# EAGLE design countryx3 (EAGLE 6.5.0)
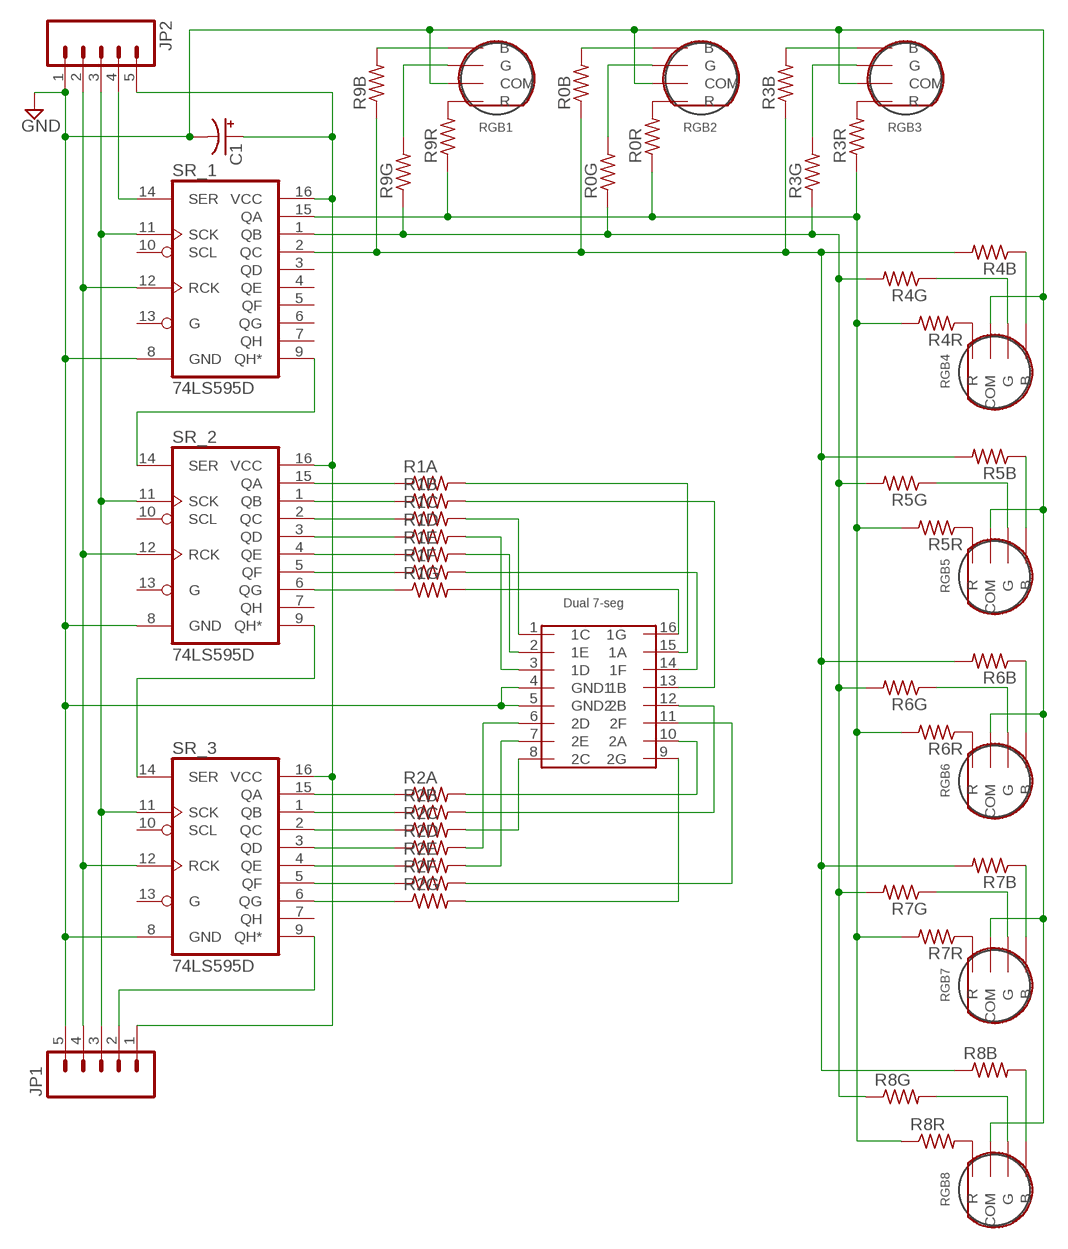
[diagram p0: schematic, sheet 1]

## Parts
C1  CPOL-USE2,5-6E  [E2,5-6E]
JP1  M05LOCK  [1X05_LOCK]
JP2  M05LOCK  [1X05_LOCK]
R0B  R-US_M0805  [M0805]
R0G  R-US_M0805  [M0805]
R0R  R-US_M0805  [M0805]
R1A  R-US_M0805  [M0805]
R1B  R-US_M0805  [M0805]
R1C  R-US_M0805  [M0805]
R1D  R-US_M0805  [M0805]
R1E  R-US_M0805  [M0805]
R1F  R-US_M0805  [M0805]
R1G  R-US_M0805  [M0805]
R2A  R-US_M0805  [M0805]
R2B  R-US_M0805  [M0805]
R2C  R-US_M0805  [M0805]
R2D  R-US_M0805  [M0805]
R2E  R-US_M0805  [M0805]
R2F  R-US_M0805  [M0805]
R2G  R-US_M0805  [M0805]
R3B  R-US_M0805  [M0805]
R3G  R-US_M0805  [M0805]
R3R  R-US_M0805  [M0805]
R4B  R-US_M0805  [M0805]
R4G  R-US_M0805  [M0805]
R4R  R-US_M0805  [M0805]
R5B  R-US_M0805  [M0805]
R5G  R-US_M0805  [M0805]
R5R  R-US_M0805  [M0805]
R6B  R-US_M0805  [M0805]
R6G  R-US_M0805  [M0805]
R6R  R-US_M0805  [M0805]
R7B  R-US_M0805  [M0805]
R7G  R-US_M0805  [M0805]
R7R  R-US_M0805  [M0805]
R8B  R-US_M0805  [M0805]
R8G  R-US_M0805  [M0805]
R8R  R-US_M0805  [M0805]
R9B  R-US_M0805  [M0805]
R9G  R-US_M0805  [M0805]
R9R  R-US_M0805  [M0805]
RGB1  RGBLED  [3LED]
RGB2  RGBLED  [3LED]
RGB3  RGBLED  [3LED]
RGB4  RGBLED  [3LED]
RGB5  RGBLED  [3LED]
RGB6  RGBLED  [3LED]
RGB7  RGBLED  [3LED]
RGB8  RGBLED  [3LED]
SR_1  74LS595D  [SO16]
SR_2  74LS595D  [SO16]
SR_3  74LS595D  [SO16]
U$1  HDSP-G03E  [HDSP-G]

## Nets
GND: C1.- JP1.5 JP2.1 RGB1.COM RGB2.COM RGB3.COM RGB4.COM RGB5.COM RGB6.COM RGB7.COM RGB8.COM SR_1.8(GND) SR_2.8(GND) SR_3.8(GND) U$1.4(GND1) U$1.5(GND2)
N$1: R0R.1 R3R.1 R4R.2 R5R.2 R6R.2 R7R.2 R8R.1 R9R.1 SR_1.15(QA)
N$2: R0B.1 R3B.1 R4B.2 R5B.2 R6B.2 R7B.2 R8B.1 R9B.1 SR_1.2(QC)
N$3: R8R.2 RGB8.R
N$4: R1G.2 U$1.16(1G)
N$5: R1F.2 U$1.14(1F)
N$6: R1C.2 U$1.1(1C)
N$7: R1G.1 SR_2.6(QG)
N$8: R9R.2 RGB1.R
N$9: R1A.2 U$1.15(1A)
N$10: R1B.2 U$1.13(1B)
N$11: R2B.2 U$1.12(2B)
N$12: R2F.2 U$1.11(2F)
N$13: R2B.1 SR_3.1(QB)
N$14: R2D.2 U$1.6(2D)
N$15: R2A.1 SR_3.15(QA)
N$16: R1D.1 SR_2.3(QD)
N$17: R2E.2 U$1.7(2E)
N$18: R0R.2 RGB2.R
N$19: R2C.1 SR_3.2(QC)
N$20: R3R.2 RGB3.R
N$21: R2A.2 U$1.10(2A)
N$22: R2D.1 SR_3.3(QD)
N$23: R2E.1 SR_3.4(QE)
N$24: R2F.1 SR_3.5(QF)
N$25: R9G.2 RGB1.G
N$26: R0G.2 RGB2.G
N$27: R3G.2 RGB3.G
N$28: R9B.2 RGB1.B
N$29: R0B.2 RGB2.B
N$30: R3B.2 RGB3.B
N$31: R2G.1 SR_3.6(QG)
N$32: R0G.1 R3G.1 R4G.2 R5G.2 R6G.2 R7G.2 R8G.1 R9G.1 SR_1.1(QB)
N$33: R1E.1 SR_2.4(QE)
N$34: R4G.1 RGB4.G
N$35: R4B.1 RGB4.B
N$36: R4R.1 RGB4.R
N$37: R2G.2 U$1.9(2G)
N$38: R1E.2 U$1.2(1E)
N$39: R5G.1 RGB5.G
N$40: R5B.1 RGB5.B
N$41: R5R.1 RGB5.R
N$42: R1F.1 SR_2.5(QF)
N$43: R6G.1 RGB6.G
N$44: R6B.1 RGB6.B
N$45: R6R.1 RGB6.R
N$46: R8G.2 RGB8.G
N$47: R8B.2 RGB8.B
N$48: R1D.2 U$1.3(1D)
N$49: R7G.1 RGB7.G
N$50: R7B.1 RGB7.B
N$51: R7R.1 RGB7.R
N$52: R2C.2 U$1.8(2C)
N$53: R1C.1 SR_2.2(QC)
N$54: R1B.1 SR_2.1(QB)
N$55: R1A.1 SR_2.15(QA)
RCLK: JP1.4 JP2.2 SR_1.12(RCK) SR_2.12(RCK) SR_3.12(RCK)
SCLK: JP1.3 JP2.3 SR_1.11(SCK) SR_2.11(SCK) SR_3.11(SCK)
SER_12: SR_1.9(QH*) SR_2.14(SER)
SER_23: SR_2.9(QH*) SR_3.14(SER)
SER_IN: JP2.4 SR_1.14(SER)
SER_OUT: JP1.2 SR_3.9(QH*)
VCC: C1.+ JP1.1 JP2.5 SR_1.16(VCC) SR_2.16(VCC) SR_3.16(VCC)
Unconnected: SR_1.3(QD) SR_1.4(QE) SR_1.5(QF) SR_1.6(QG) SR_1.7(QH) SR_1.10(SCL) SR_1.13(G) SR_2.7(QH) SR_2.10(SCL) SR_2.13(G) SR_3.7(QH) SR_3.10(SCL) SR_3.13(G)

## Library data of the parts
C1 = Power Supply:CPOL-US: POLARIZED CAPACITOR, American symbol
JP1 JP2 = SparkFun-Connectors:M05: Header 5 Standard 5-pin 0.1" header. Use with straight break away headers (SKU : PRT-00116), right angle break away headers (PRT-00553), swiss pins (PRT-00743), machine pins (PRT-00117), and female headers (PRT-00115). Molex polarized connector foot print use with SKU : PRT-08230 with associated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
R0B R0G R0R R1A R1B R1C R1D R1E R1F R1G R2A R2B R2C R2D R2E R2F R2G R3B R3G R3R R4B R4G R4R R5B R5G R5R R6B R6G R6R R7B R7G R7R R8B R8G R8R R9B R9G R9R = resistor:R-US_: RESISTOR, American symbol
RGB1-RGB8 = RISK:RGBLED
SR_1-SR_3 = SparkFun-DigitalIC:74*595: 8-bit SHIFT REGISTER, output latch; PROD_ID: IC-07875
U$1 = RISK:HDSP-G03E

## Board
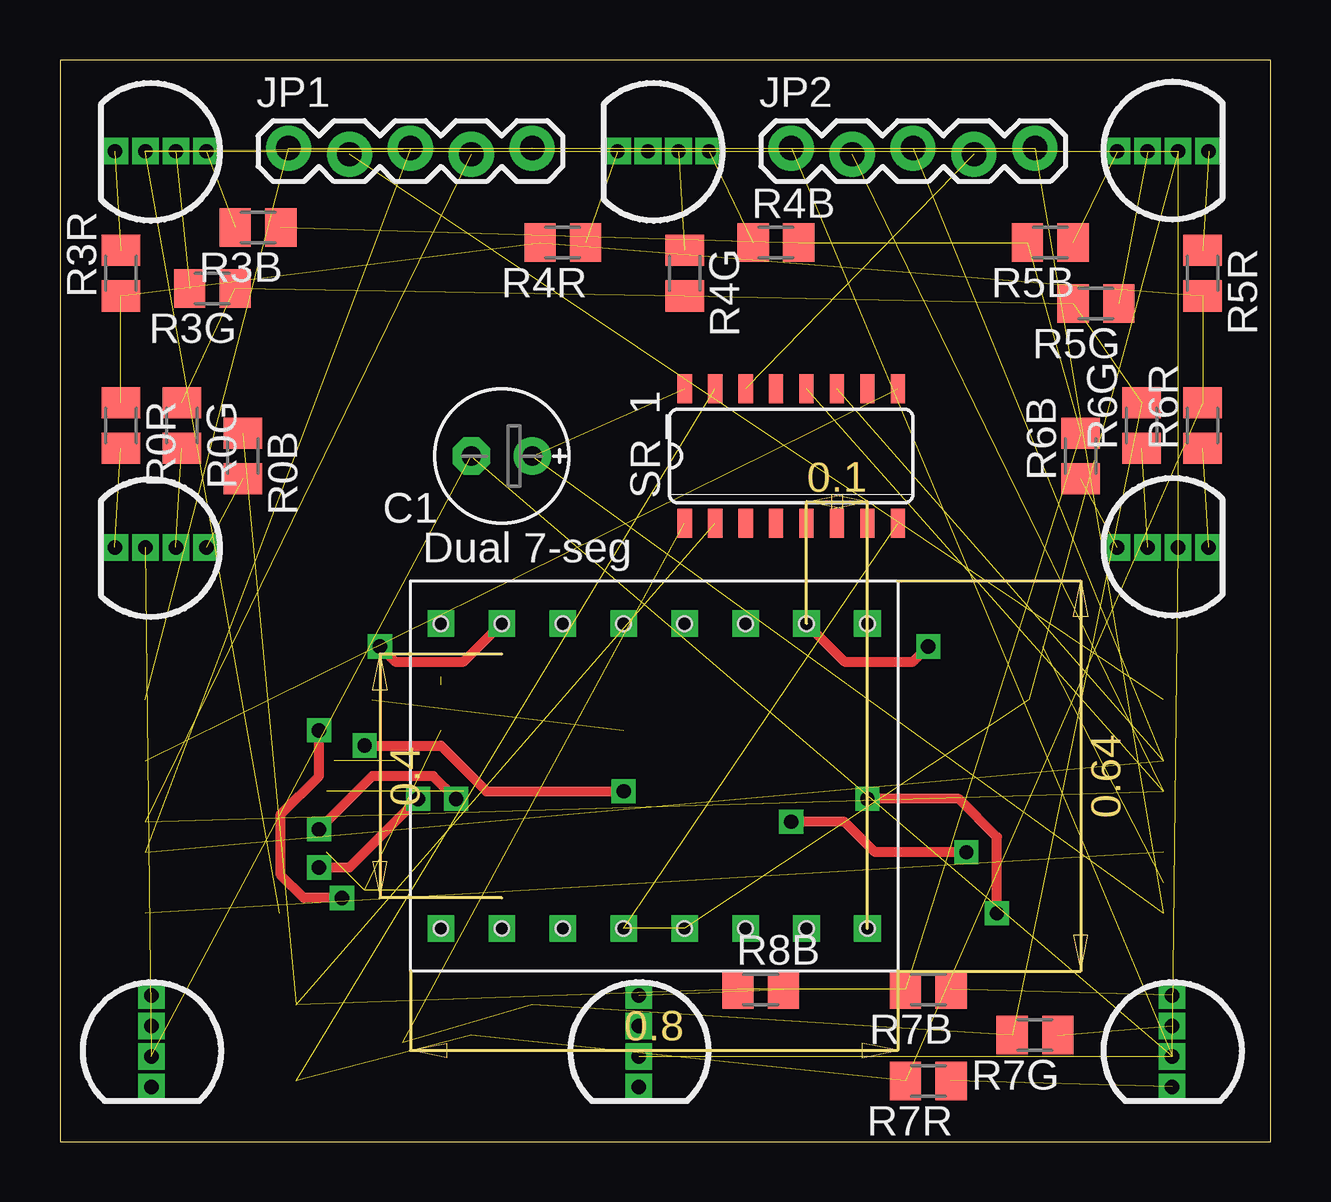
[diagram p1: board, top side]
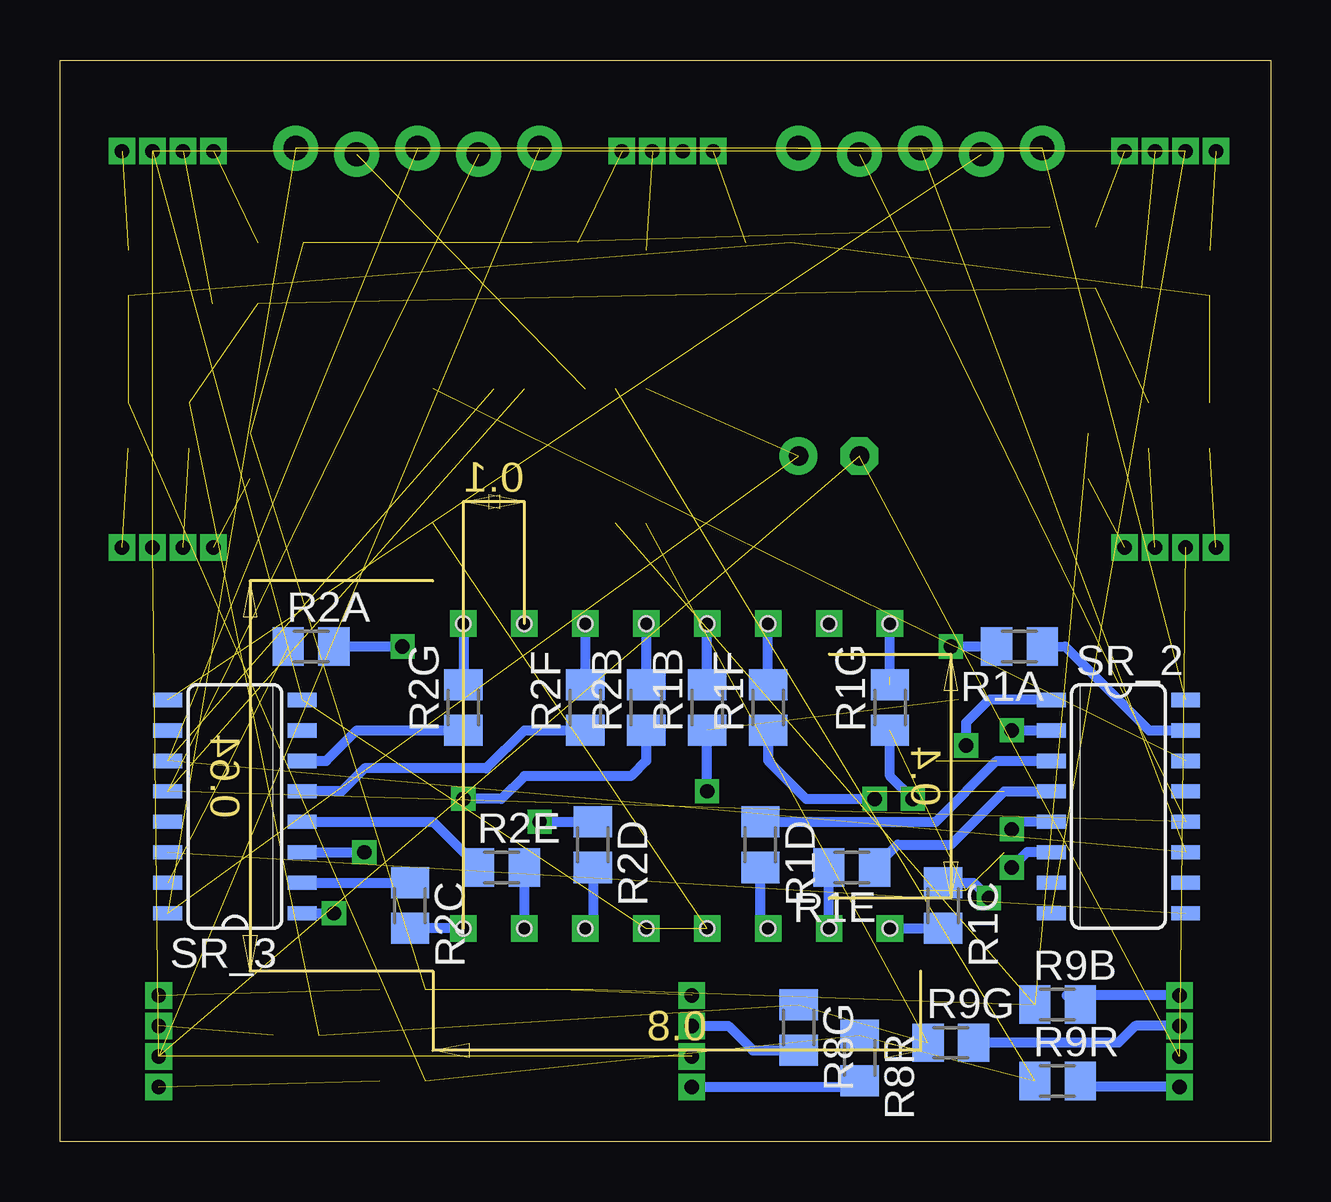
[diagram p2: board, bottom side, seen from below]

Size 50.47 x 45.08 mm. Coordinates in mm from the lower left corner, seen from the top.
Outline: 0,0 50.47,0 50.47,45.08 0,45.08 0,0
Copper layers (1*16): Top 0.035mm / dielectric 1.5mm / Bottom 0.035mm
Design rules "default": minimum track width 10mil, minimum drill 24mil, track to track 8mil, track to pad 8mil, pad to pad 8mil, via to via 8mil, smd to smd 8mil, copper to edge 40mil, drill to drill 8mil, minimum pad ring 10mil, minimum via ring 8mil, stop-mask expansion 4mil, vias tented up to drill 0mil, thermal gap 10mil

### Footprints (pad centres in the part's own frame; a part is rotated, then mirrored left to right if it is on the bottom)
E2,5-6E = drill 0.813 pad 1.575: + -1.27,0 | drill 0.813 pad 1.575 octagon: - 1.27,0
1X05_LOCK = drill 1.016 pad 1.88: 1 0,0.127; 2 2.54,-0.127; 3 5.08,0.127; 4 7.62,-0.127; 5 10.16,0.127
M0805 = smd 1.3 x 1.6: 1 -0.95,0; 2 0.95,0
3LED = drill 0.6 pad 0.61 square: B 0,2.286; COM 0,-0.254; G 0,1.016; R 0,-1.524
SO16 = smd 0.6 x 1.2: 1 -4.445,-2.8; 2 -3.175,-2.8; 3 -1.905,-2.8; 4 -0.635,-2.8; 5 0.635,-2.8; 6 1.905,-2.8; 7 3.175,-2.8; 8 4.445,-2.8; 9 4.445,2.8; 10 3.175,2.8; 11 1.905,2.8; 12 0.635,2.8; 13 -0.635,2.8; 14 -1.905,2.8; 15 -3.175,2.8; 16 -4.445,2.8
HDSP-G = drill 0.6 square: 1 -8.89,-6.35; 2 -6.35,-6.35; 3 -3.81,-6.35; 4 -1.27,-6.35; 5 1.27,-6.35; 6 3.81,-6.35; 7 6.35,-6.35; 8 8.89,-6.35; 9 8.89,6.35; 10 6.35,6.35; 11 3.81,6.35; 12 1.27,6.35; 13 -1.27,6.35; 14 -3.81,6.35; 15 -6.35,6.35; 16 -8.89,6.35 | hole 0.6: 1.27,-6.35; 1.27,-6.35; 1.27,-6.35; 1.27,-6.35; -1.27,-6.35; -1.27,-6.35; -3.81,-6.35; -3.81,-6.35; -6.35,-6.35; -6.35,-6.35; -6.35,-6.35; -8.89,-6.35; -8.89,-6.35; 3.81,-6.35; 3.81,-6.35; 3.81,-6.35; 6.35,-6.35; 6.35,-6.35; 8.89,-6.35; 8.89,-6.35; 8.89,-6.35; 8.89,6.35; 8.89,6.35; 6.35,6.35; 6.35,6.35; 3.81,6.35; 3.81,6.35; 1.27,6.35; 1.27,6.35; -1.27,6.35; -1.27,6.35; -3.81,6.35; -3.81,6.35; -6.35,6.35; -6.35,6.35; -6.35,6.35; -8.89,6.35; -8.89,6.35

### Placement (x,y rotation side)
C1  18.41,28.57 180 top
JP1  9.53,41.27 0 top
JP2  30.48,41.27 0 top
R0B  7.62,28.57 270 top
R0G  5.08,29.84 270 top
R0R  2.54,29.84 270 top
R1A  10.48,20.64 180 bottom
R1B  23.5,18.1 90 bottom
R1C  13.65,9.84 270 bottom
R1D  21.27,12.38 270 bottom
R1E  17.46,11.43 180 bottom
R1F  20.95,18.1 90 bottom
R1G  15.88,18.1 90 bottom
R2A  40.01,20.64 0 bottom
R2B  26.04,18.1 90 bottom
R2C  35.88,9.84 270 bottom
R2D  28.26,12.38 270 bottom
R2E  32.07,11.43 0 bottom
R2F  28.57,18.1 90 bottom
R2G  33.66,18.1 90 bottom
R3B  8.26,38.1 180 top
R3G  6.35,35.56 180 top
R3R  2.54,36.2 90 top
R4B  29.84,37.47 0 top
R4G  26.04,36.2 270 top
R4R  20.95,37.47 180 top
R5B  41.27,37.47 180 top
R5G  43.18,34.92 180 top
R5R  47.62,36.2 270 top
R6B  42.55,28.57 90 top
R6G  45.09,29.84 90 top
R6R  47.62,29.84 90 top
R7B  36.2,6.35 180 top
R7G  40.64,4.45 180 top
R7R  36.2,2.54 180 top
R8B  29.21,6.35 0 top
R8G  19.68,4.76 270 bottom
R8R  17.14,3.49 270 bottom
R9B  8.89,5.71 0 bottom
R9G  13.34,4.13 0 bottom
R9R  8.89,2.54 0 bottom
RGB1  3.81,3.81 0 top
RGB2  3.81,24.77 270 top
RGB3  3.81,41.27 270 top
RGB4  24.77,41.27 270 top
RGB5  46.35,41.27 90 top
RGB6  46.35,24.77 90 top
RGB7  46.35,3.81 0 top
RGB8  24.13,3.81 0 top
SR_1  30.48,28.57 0 top
SR_2  6.35,13.97 270 bottom
SR_3  43.18,13.97 90 bottom
U$1  24.77,15.24 0 top

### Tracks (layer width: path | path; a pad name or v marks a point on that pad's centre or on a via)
GND  (15 unrouted)
N$1  (8 unrouted)
N$2  (8 unrouted)
N$3
  Bottom 0.406: RGB8.R 17.4,2.29 R8R.2
N$4  (1 unrouted)
  Bottom 0.406: 15.88,19.37 U$1.16
N$5
  Bottom 0.406: R1F.2 U$1.14
N$6
  Bottom 0.406: U$1.1 13.97,8.89 R1C.2
N$7  (via drill 0.6)  (3 unrouted)
  Top 0.406: v10.79,11.43 12.06,11.43 v14.92,14.29
  Bottom 0.406: SR_2.6 10.16,12.06 v10.79,11.43 | v14.92,14.29 15.88,15.24 R1G.1
N$8
  Bottom 0.406: RGB1.R 8.32,2.29 R9R.2
N$9  (via drill 0.6)
  Top 0.406: v13.34,20.64 13.97,20 16.83,20 U$1.15
  Bottom 0.406: R1A.2 v13.34,20.64
N$10
  Bottom 0.406: R1B.2 U$1.13
N$11
  Bottom 0.406: U$1.12 R2B.2
N$12
  Bottom 0.406: U$1.11 R2F.2
N$13  (via drill 0.6)
  Top 0.406: v39.05,9.53 39.05,12.7 37.47,14.29 v33.66,14.29
  Bottom 0.406: R2B.1 26.04,15.88 26.67,15.24 31.11,15.24 32.07,14.29 v33.66,14.29 | SR_3.1 v39.05,9.53
N$14
  Bottom 0.406: R2D.2 28.26,9.21 U$1.6
N$15  (1 unrouted)
N$16  (1 unrouted)
  Bottom 0.406: R1D.1 20.32,13.33 16.51,13.34 13.97,13.34 11.43,15.88 SR_2.3
N$17
  Bottom 0.406: U$1.7 R2E.2
N$18  (1 unrouted)
N$19
  Bottom 0.406: SR_3.2 R2C.1
N$20  (1 unrouted)
N$21  (via drill 0.6)
  Top 0.406: U$1.10 32.7,20 35.56,20 v36.2,20.64
  Bottom 0.406: v36.2,20.64 R2A.2
N$22  (via drill 0.6)
  Top 0.406: v37.78,12.06 33.97,12.06 32.7,13.34 v30.48,13.34
  Bottom 0.406: SR_3.3 v37.78,12.06 | v30.48,13.34 R2D.1
N$23
  Bottom 0.406: SR_3.4 34.92,13.34 R2E.1
N$24
  Bottom 0.406: SR_3.5 38.73,14.61 37.78,15.56 32.7,15.56 31.11,17.14 R2F.1
N$25
  Bottom 0.406: RGB1.G 5.65,4.83 6.35,4.13 R9G.2
N$26  (1 unrouted)
N$27  (1 unrouted)
N$28
  Bottom 0.406: RGB1.B 8.51,6.1 R9B.2
N$29  (1 unrouted)
N$30  (1 unrouted)
N$31
  Bottom 0.406: SR_3.6 39.37,15.88 38.1,17.14 34.29,17.14 R2G.1
N$32  (8 unrouted)
N$33  (1 unrouted)
  Bottom 0.406: SR_2.4 11.11,14.61 13.34,12.38 15.56,12.38 16.2,11.74 R1E.1
N$34  (1 unrouted)
N$35  (1 unrouted)
N$36  (1 unrouted)
N$37
  Bottom 0.406: U$1.9 R2G.2
N$38
  Bottom 0.406: U$1.2 18.41,11.11 R1E.2
N$39  (1 unrouted)
N$40  (1 unrouted)
N$41  (1 unrouted)
N$42  (via drill 0.6)
  Top 0.406: v10.79,13.02 13.02,15.24 15.56,15.24 v16.51,14.29
  Bottom 0.406: SR_2.5 10.48,13.34 v10.79,13.02 | R1F.1 20.96,15.88 19.37,14.29 v16.51,14.29
N$43  (1 unrouted)
N$44  (1 unrouted)
N$45  (1 unrouted)
N$46
  Bottom 0.406: RGB8.G 22.61,4.83 21.59,3.81 R8G.2
N$47  (1 unrouted)
N$48
  Bottom 0.406: U$1.3 21.27,9.21 R1D.2
N$49  (1 unrouted)
N$50  (1 unrouted)
N$51  (1 unrouted)
N$52
  Bottom 0.406: U$1.8 R2C.2
N$53  (via drill 0.6)
  Top 0.406: v11.75,10.16 10.16,10.16 9.21,11.11 9.21,13.65 10.79,15.24 v10.79,17.14
  Bottom 0.406: R1C.1 12.38,10.79 v11.75,10.16 | v10.79,17.14 SR_2.2
N$54  (via drill 0.6)  (1 unrouted)
  Top 0.406: v12.7,16.51 15.88,16.51 17.78,14.61 v23.5,14.61
  Bottom 0.406: SR_2.1 11.75,18.41 12.7,17.46 v12.7,16.51 | v23.5,14.61 R1B.1
N$55
  Bottom 0.406: SR_2.15 5.08,17.14 8.57,20.64 R1A.1
RCLK  (4 unrouted)
SCLK  (4 unrouted)
SER_12  (1 unrouted)
SER_23  (1 unrouted)
SER_IN  (1 unrouted)
SER_OUT  (1 unrouted)
VCC  (5 unrouted)

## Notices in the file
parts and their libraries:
SparkFun-DigitalIC: Licensing: Creative Commons ShareAlike 4.0 International - https://creativecommons.org/licenses/by-sa/4.0
